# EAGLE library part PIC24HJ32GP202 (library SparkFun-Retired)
PIC24HJ32GP202 Retired: IC-08923
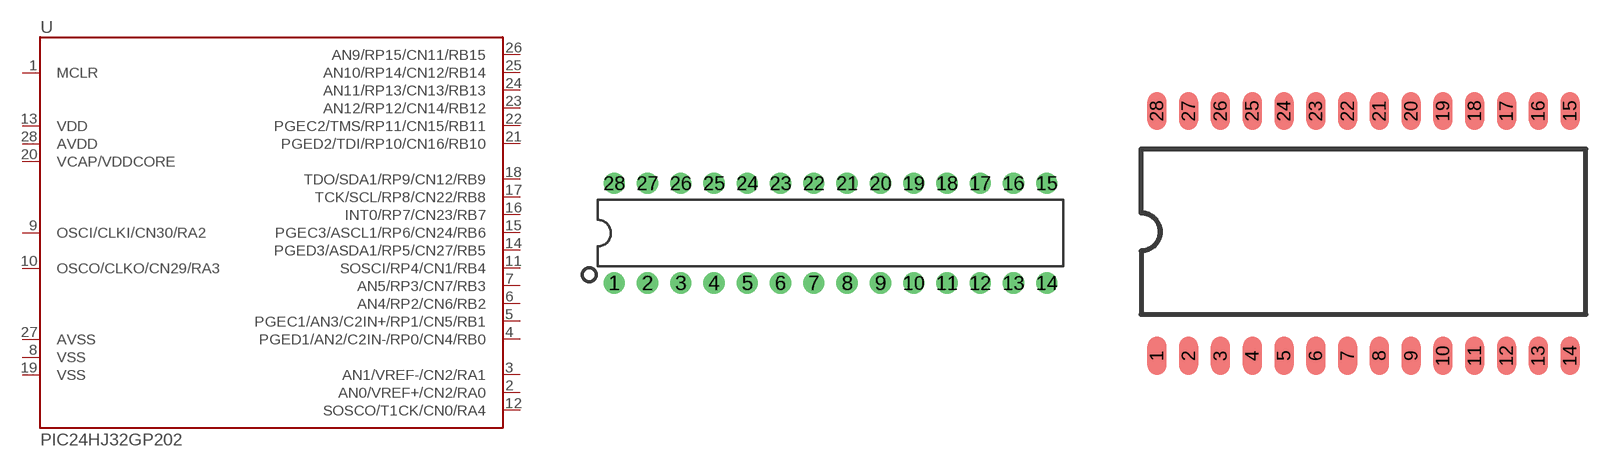
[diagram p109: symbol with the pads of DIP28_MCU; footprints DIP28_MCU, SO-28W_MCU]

Designator prefix -

## PIC24HJ32GP202DIP  [DIP28_MCU]
1  MCLR  in
2  AN0/VREF+/CN2/RA0
3  AN1/VREF-/CN2/RA1
4  PGED1/AN2/C2IN-/RP0/CN4/RB0
5  PGEC1/AN3/C2IN+/RP1/CN5/RB1
6  AN4/RP2/CN6/RB2
7  AN5/RP3/CN7/RB3
8  VSS  pwr
9  OSCI/CLKI/CN30/RA2  in
10  OSCO/CLKO/CN29/RA3  out
11  SOSCI/RP4/CN1/RB4
12  SOSCO/T1CK/CN0/RA4
13  VDD  pwr
14  PGED3/ASDA1/RP5/CN27/RB5
15  PGEC3/ASCL1/RP6/CN24/RB6
16  INT0/RP7/CN23/RB7
17  TCK/SCL/RP8/CN22/RB8
18  TDO/SDA1/RP9/CN12/RB9
19  VSS  pwr
20  VCAP/VDDCORE  pwr
21  PGED2/TDI/RP10/CN16/RB10
22  PGEC2/TMS/RP11/CN15/RB11
23  AN12/RP12/CN14/RB12
24  AN11/RP13/CN13/RB13
25  AN10/RP14/CN12/RB14
26  AN9/RP15/CN11/RB15
27  AVSS  pwr
28  AVDD  pwr

## PIC24HJ32GP202SMD  [SO-28W_MCU]
Pads as for DIP28_MCU

## Footprint DIP28_MCU (pad centres in mm)
Standard 28-pin DIP package. IC needs to have legs bent before insertion.
drill 0.813 pad 1.626: 1 -16.51,-3.81; 2 -13.97,-3.81; 3 -11.43,-3.81; 4 -8.89,-3.81; 5 -6.35,-3.81; 6 -3.81,-3.81; 7 -1.27,-3.81; 8 1.27,-3.81; 9 3.81,-3.81; 10 6.35,-3.81; 11 8.89,-3.81; 12 11.43,-3.81; 13 13.97,-3.81; 14 16.51,-3.81; 15 16.51,3.81; 16 13.97,3.81; 17 11.43,3.81; 18 8.89,3.81; 19 6.35,3.81; 20 3.81,3.81; 21 1.27,3.81; 22 -1.27,3.81; 23 -3.81,3.81; 24 -6.35,3.81; 25 -8.89,3.81; 26 -11.43,3.81; 27 -13.97,3.81; 28 -16.51,3.81

## Footprint SO-28W_MCU (pad centres in mm)
Small Outline Wide Plastic Gull Wing 300-mil body, package type SO
smd 0.762 x 1.524: 1 -8.255,-4.953; 2 -6.985,-4.953; 3 -5.715,-4.953; 4 -4.445,-4.953; 5 -3.175,-4.953; 6 -1.905,-4.953; 7 -0.635,-4.953; 8 0.635,-4.953; 9 1.905,-4.953; 10 3.175,-4.953; 11 4.445,-4.953; 12 5.715,-4.953; 13 6.985,-4.953; 14 8.255,-4.953; 15 8.255,4.826; 16 6.985,4.826; 17 5.715,4.826; 18 4.445,4.826; 19 3.175,4.826; 20 1.905,4.826; 21 0.635,4.826; 22 -0.635,4.826; 23 -1.905,4.826; 24 -3.175,4.826; 25 -4.445,4.826; 26 -5.715,4.826; 27 -6.985,4.826; 28 -8.255,4.826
